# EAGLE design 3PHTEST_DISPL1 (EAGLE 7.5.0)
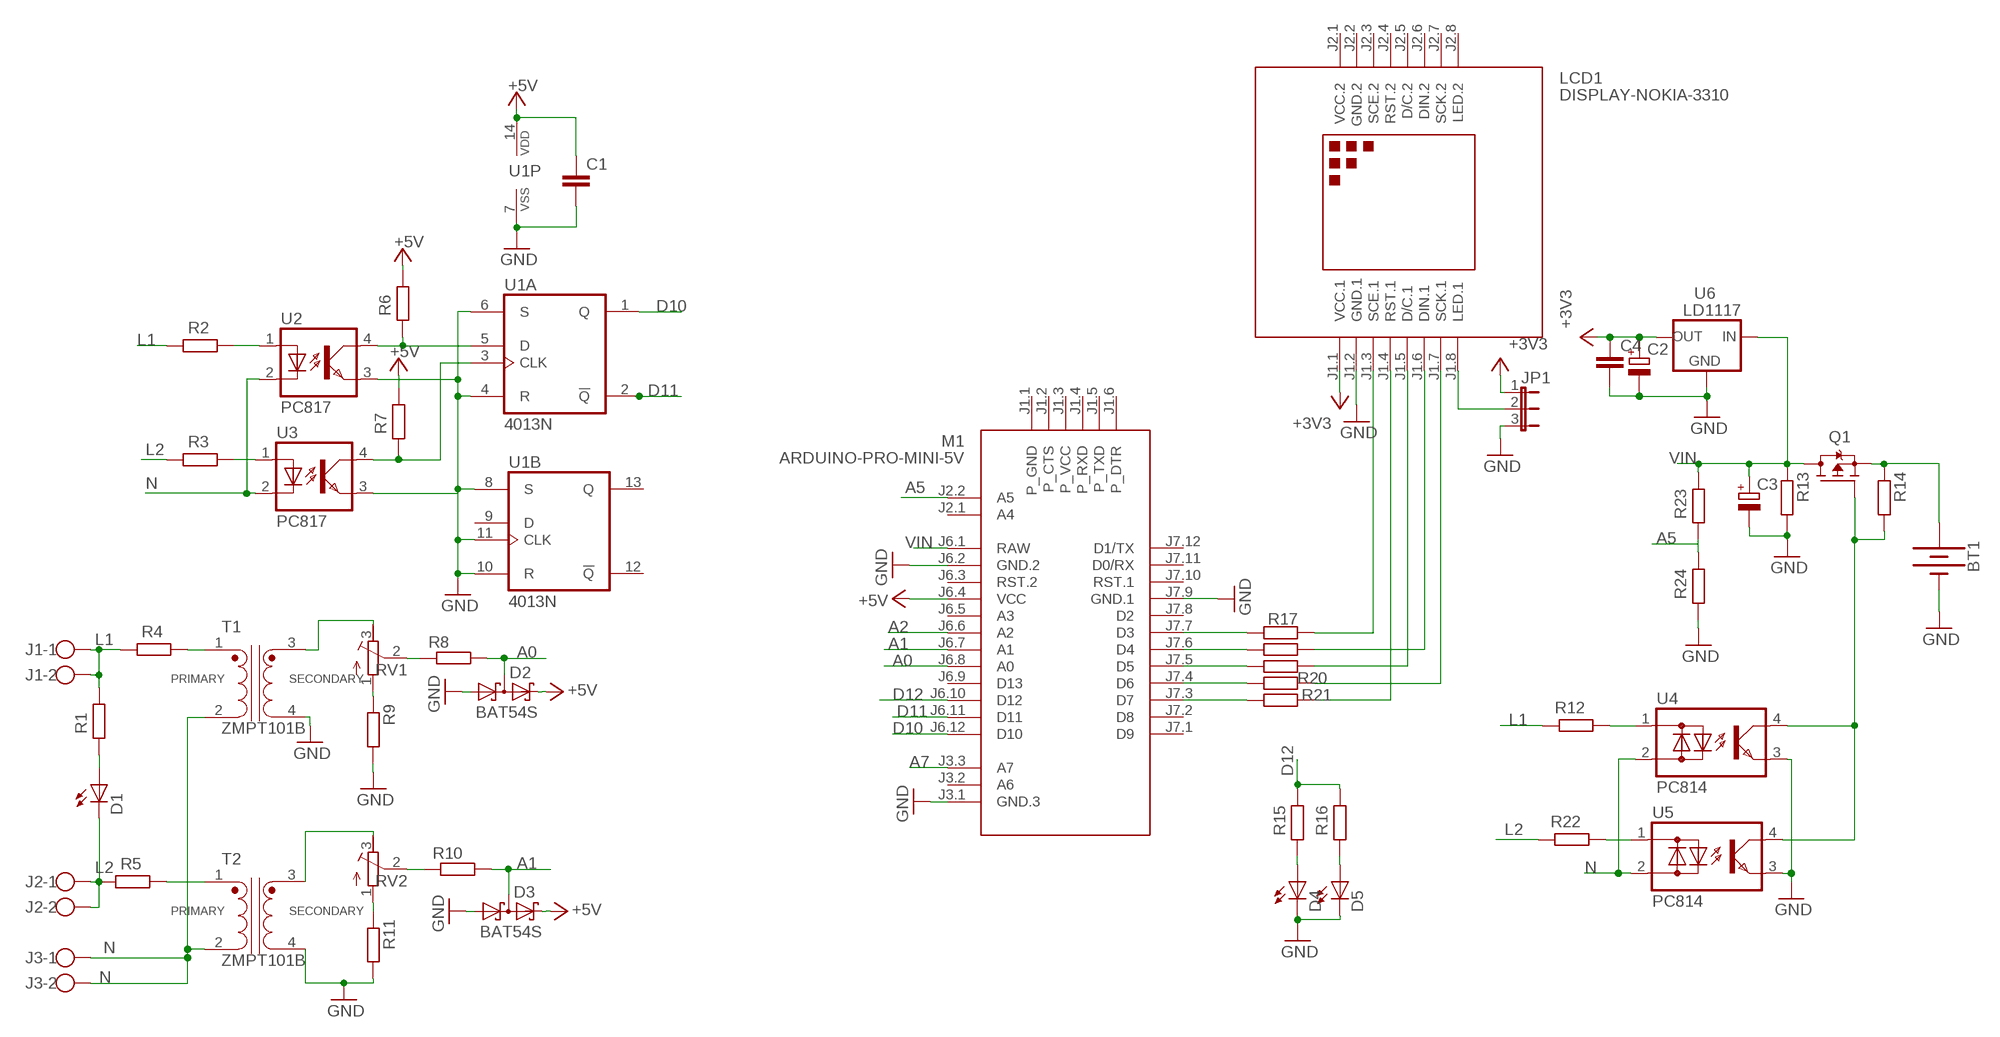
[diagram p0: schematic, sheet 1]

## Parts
BT1  BATTERY-9V  [BATTCON_9V]
C1  C-EUC1206  [C1206]
C2  CPOL-EUSMCB  [SMC_B]
C3  CPOL-EUSMCB  [SMC_B]
C4  C-EUC1206  [C1206]
D1  LED5MM  [LED5MM]
D2  BAT54S  [SOT23]
D3  BAT54S  [SOT23]
D4  LED5MM  [LED5MM]
D5  LED5MM  [LED5MM]
J1  W237-102  [W237-102]
J2  W237-102  [W237-102]
J3  W237-102  [W237-102]
JP1  JP2E  [JP2]
LCD1  DISPLAY-NOKIA-3310  [DISPLAY-NOKIA-3310]
M1  ARDUINO-PRO-MINI-5V  ARDUINO-PRO-MINI-3.3V  [ARDUINO-PRO-MINI]
Q1  STR2P3LLH6  [SOT23]
R1  R-EU_R2512  [R2512]
R2  R-EU_R2512  [R2512]
R3  R-EU_R2512  [R2512]
R4  R-EU_R2512  [R2512]
R5  R-EU_R2512  [R2512]
R6  R-EU_R1206  [R1206]
R7  R-EU_R1206  [R1206]
R8  R-EU_R1206  [R1206]
R9  R-EU_R1206  [R1206]
R10  R-EU_R1206  [R1206]
R11  R-EU_R1206  [R1206]
R12  R-EU_R2512  [R2512]
R13  R-EU_R1206  [R1206]
R14  R-EU_R1206  [R1206]
R15  R-EU_R1206  [R1206]
R16  R-EU_R1206  [R1206]
R17  R-EU_R1206  [R1206]
R18  R-EU_R1206  [R1206]
R19  R-EU_R1206  [R1206]
R20  R-EU_R1206  [R1206]
R21  R-EU_R1206  [R1206]
R22  R-EU_R2512  [R2512]
R23  R-EU_R1206  [R1206]
R24  R-EU_R1206  [R1206]
RV1  R-TRIMM64W  [RTRIM64W]
RV2  R-TRIMM64W  [RTRIM64W]
T1  ZMPT101B  [XFMR_ZMPT101B]
T2  ZMPT101B  [XFMR_ZMPT101B]
U1  4013N  [DIL14]
U2  PC817  [DIL04]
U3  PC817  [DIL04]
U4  PC814  [DIL04]
U5  PC814  [DIL04]
U6  LD1117  [SOT223]

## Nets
+3V3: C2.+ C4.1 JP1.1 LCD1.J1.1(VCC.1) U6.2(OUT)
+5V: C1.1 D2.2(C2) D3.2(C2) M1.J6.4(VCC) R6.1 R7.1 U1.14(P:VDD)
A0: D2.3(C1A2) M1.J6.8(A0) R8.2
A1: D3.3(C1A2) M1.J6.7(A1) R10.2
A2: M1.J6.6(A2)
A5: M1.J2.2(A5) R23.2 R24.1
A7: M1.J3.3(A7)
D10: M1.J6.12(D10) U1.1(A:Q)
D11: M1.J6.11(D11) U1.2(A:!Q)
D12: M1.J6.10(D12) R15.1 R16.1
GND: BT1.- C1.2 C2.- C3.- C4.2 D2.1(A1) D3.1(A1) D4.K(C) D5.K(C) JP1.3 LCD1.J1.2(GND.1) M1.J3.1(GND.3) M1.J6.2(GND.2) M1.J7.9(GND.1) R9.2 R11.2 R13.2 R24.2 T1.4 T2.4 U1.4(A:R) U1.6(A:S) U1.7(P:VSS) U1.8(B:S) U1.10(B:R) U1.11(B:CLK) U2.3(EMIT) U3.3(EMIT) U4.3(E) U5.3(E) U6.1(GND)
L1: J1.1 J1.2 R1.1 R2.2 R4.2 R12.2
L2: D1.K(C) J2.1 J2.2 R3.2 R5.2 R22.2
N: J3.1 J3.2 T1.2 T2.2 U2.2(C) U3.2(C) U4.2(AC2) U5.2(AC2)
N$1: BT1.+ Q1.3(S) R14.1
N$2: Q1.2(G) R14.2 U4.4(C) U5.4(C)
N$3: LCD1.J1.4(RST.1) R21.1
N$4: M1.J7.7(D3) R17.2
N$5: M1.J7.6(D4) R18.2
N$6: LCD1.J1.6(DIN.1) R18.1
N$7: M1.J7.3(D7) R21.2
N$8: LCD1.J1.7(SCK.1) R20.1
N$9: LCD1.J1.3(SCE.1) R17.1
N$10: LCD1.J1.5(D/C.1) R19.1
N$11: M1.J7.5(D5) R19.2
N$12: M1.J7.4(D6) R20.2
N$13: JP1.2 LCD1.J1.8(LED.1)
N$14: R12.1 U4.1(AC1)
N$15: R22.1 U5.1(AC1)
N$16: R9.1 RV1.1(A)
N$17: R4.1 T1.1
N$18: RV1.3(E) T1.3
N$19: R11.1 RV2.1(A)
N$20: R5.1 T2.1
N$21: RV2.3(E) T2.3
N$22: D1.A R1.2
N$23: R2.1 U2.1(A)
N$24: R3.1 U3.1(A)
N$25: R6.2 U1.5(A:D) U2.4(COL)
N$26: R7.2 U1.3(A:CLK) U3.4(COL)
N$27: D4.A R15.2
N$28: D5.A R16.2
N$29: R8.1 RV1.2(S)
N$32: R10.1 RV2.2(S)
VIN: C3.+ M1.J6.1(RAW) Q1.1(D) R13.1 R23.1 U6.3(IN)
Unconnected: LCD1.J2.3(SCE.2) LCD1.J2.4(RST.2) LCD1.J2.5(D/C.2) LCD1.J2.6(DIN.2) LCD1.J2.7(SCK.2) LCD1.J2.8(LED.2) M1.J1.1(P_GND) M1.J1.2(P_CTS) M1.J1.3(P_VCC) M1.J1.4(P_RXD) M1.J1.5(P_TXD) M1.J1.6(P_DTR) M1.J2.1(A4) M1.J3.2(A6) M1.J6.3(RST.2) M1.J6.5(A3) M1.J6.9(D13) M1.J7.1(D9) M1.J7.2(D8) M1.J7.8(D2) M1.J7.10(RST.1) M1.J7.11(D0/RX) M1.J7.12(D1/TX) U1.9(B:D) U1.12(B:!Q) U1.13(B:Q)

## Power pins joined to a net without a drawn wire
GND.2: LCD1.J2.2(GND.2)
VCC.2: LCD1.J2.1(VCC.2)

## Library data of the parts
BT1 = SparkFun-Batteries:BATTERY: Battery - Single Cell; PROD_ID: BATT-10855
C1 C4 = rcl:C-EU: CAPACITOR, European symbol
C2 C3 = rcl:CPOL-EU: POLARIZED CAPACITOR, European symbol
D1 D4 D5 = led:LED: LED
D2 D3 = diode:BAT54S: Schottky Diodes Pin connection corrected 2011-05-04 Source: Fairchild .. BAT54.pdf
J1-J3 = con-wago-500:W237-102: WAGO SCREW CLAMP; MPN: 237-102; OC_FARNELL: unknown; OC_NEWARK: 70K9898
JP1 = jumper:JP2E: JUMPER
LCD1 = diy-modules:DISPLAY-NOKIA-3310: 84x48 Dot Matrix LCD Module based on Nokia 3310 display More details available here: https://arduinoandsoftware.wordpress.com/2012/12/30/nokia-33105110-3-3v-display-with-5v-arduino/
M1 = diy-modules:ARDUINO-PRO-MINI-*: Arduino Pro Mini and compatible devices More details available here: https://www.arduino.cc/en/Main/ArduinoBoardProMini Click here to find device on ebay.com
Q1 = transistor-fet:STR2P3LLH6
R1-R24 = rcl:R-EU_: RESISTOR, European symbol
RV1 RV2 = rcl:R-TRIMM: Trimm resistor
T1 T2 = ZMPT101B:ZMPT101B: Check availability; AVAILABILITY: Not in stock; CHECK_PRICES: https://www.snapeda.com/parts/ZMPT101B/Qingxian+Zeming+Langxi+Electronic/view-part/?ref=eda; DESCRIPTION: Current-type Voltage Transformer; MF: Qingxian Zeming Langxi Electronic; MP: ZMPT101B; PACKAGE: None; PRICE: None; SNAPEDA_LINK: https://www.snapeda.com/parts/ZMPT101B/Qingxian+Zeming+Langxi+Electronic/view-part/?ref=snap
U1 = 40xx:4013: Dual D FLIP FLOP, set/reset
U2 U3 = optocoupler:PC817: SHARP OPTO COUPLER; MPN: PC817X4J000F; OC_FARNELL: 9707727; OC_NEWARK: 97K7059
U4 U5 = optocoupler:PC814: SHARP OPTO COUPLER; OC_FARNELL: 9707662; OC_NEWARK: unknown
U6 = v-reg:LD1117

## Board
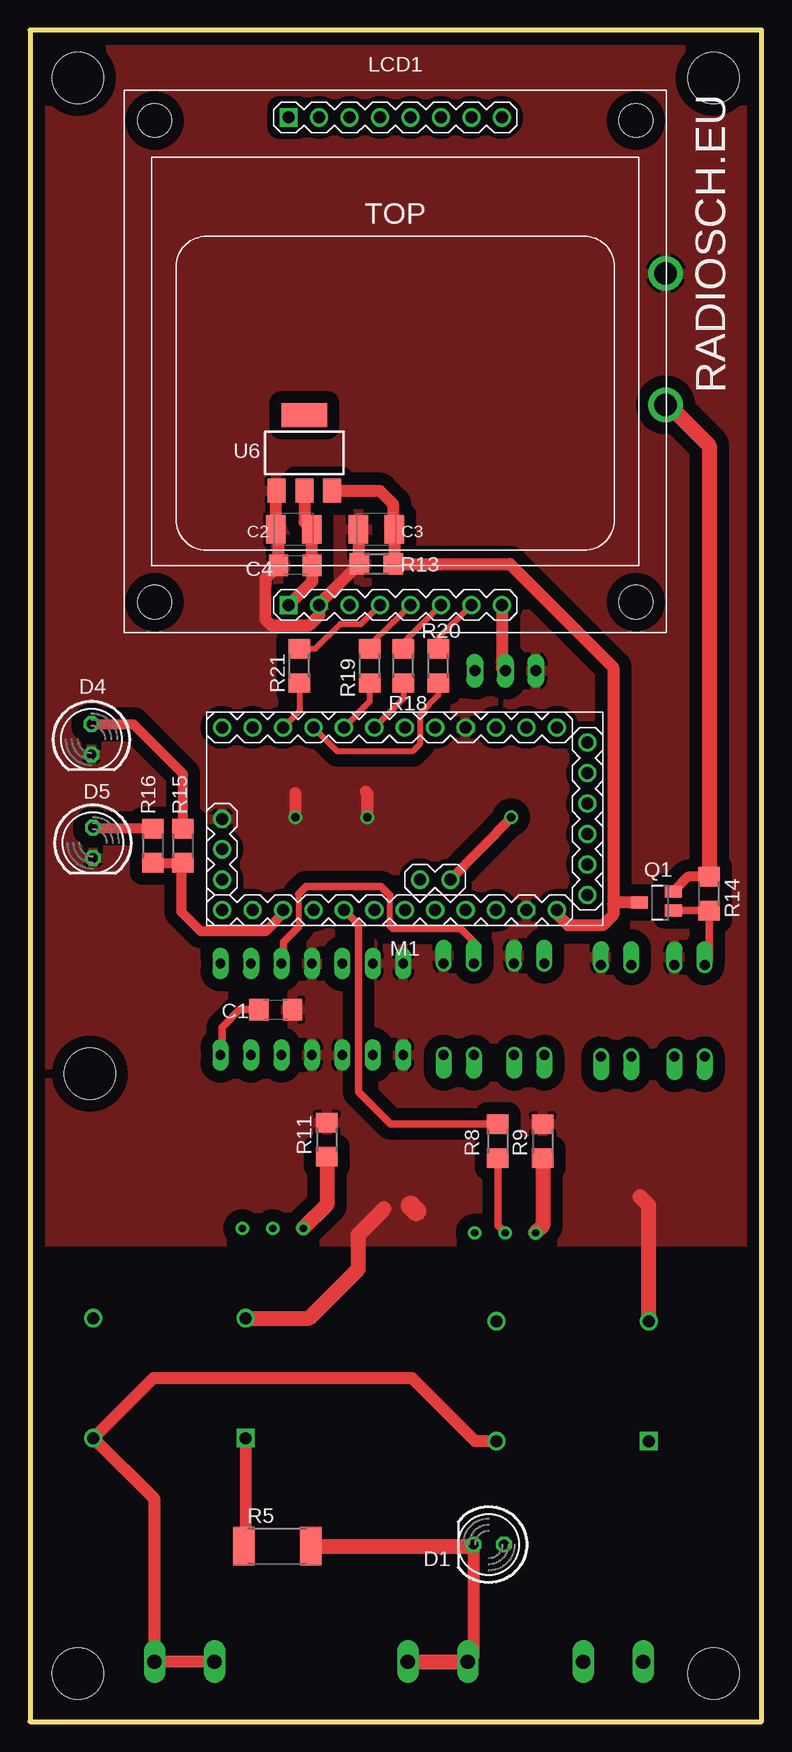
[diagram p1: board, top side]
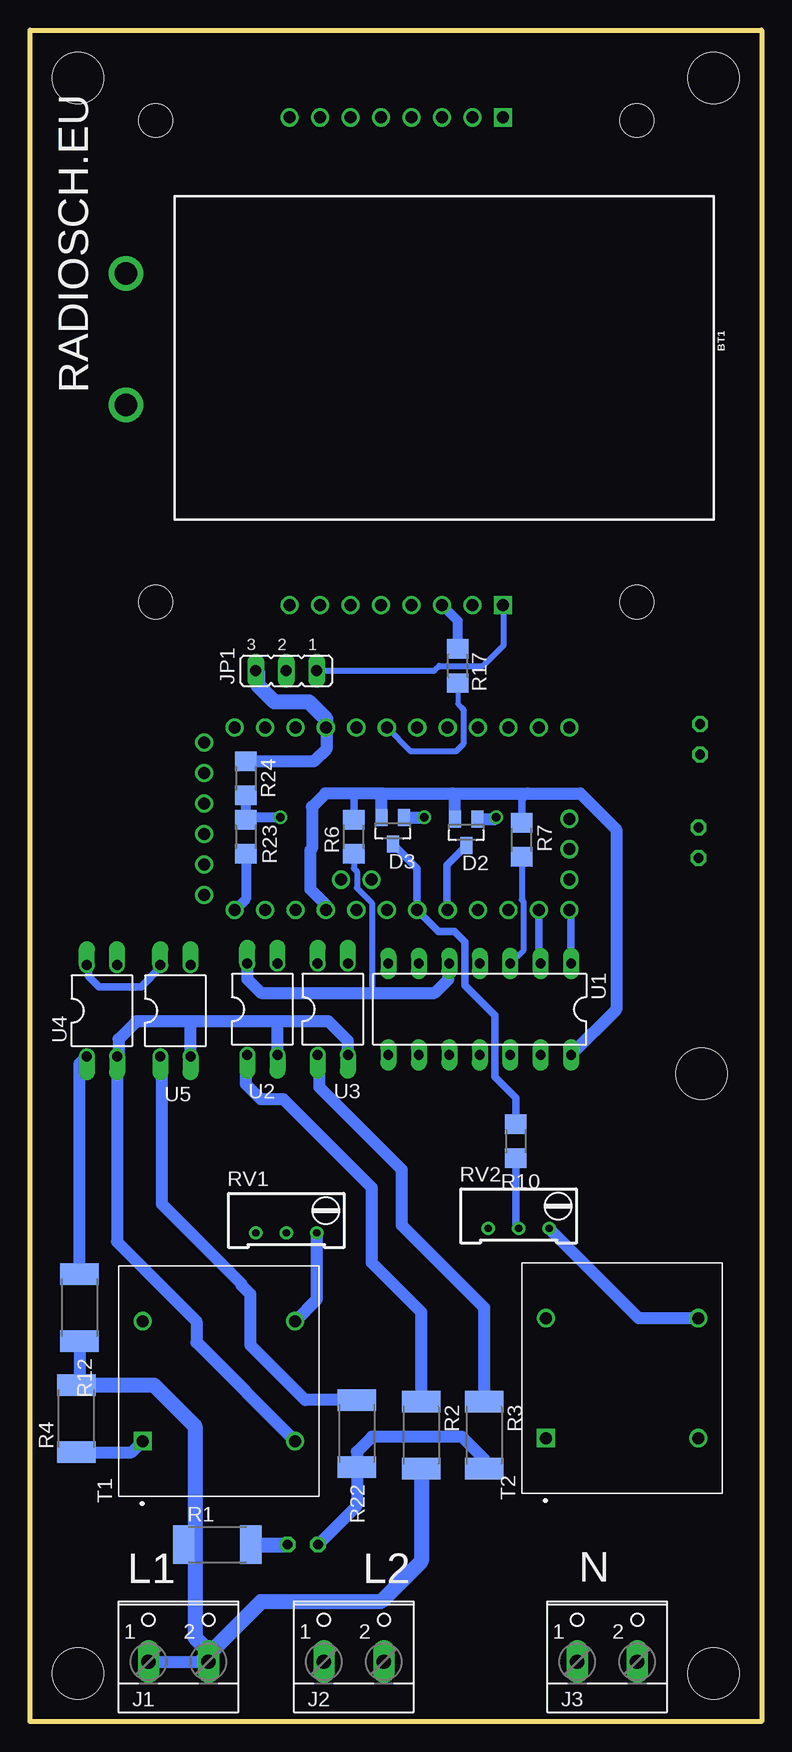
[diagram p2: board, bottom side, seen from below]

Size 61 x 141 mm. Coordinates in mm from the lower left corner, seen from the top.
Outline: 0,0 61,0 61,141 0,141 0,0
Copper layers (1*16): Top 0.035mm / dielectric 1.5mm / Bottom 0.035mm
Design rules "default": minimum track width 10mil, minimum drill 24mil, track to track 8mil, track to pad 8mil, pad to pad 8mil, via to via 8mil, smd to smd 8mil, copper to edge 40mil, drill to drill 8mil, minimum pad ring 10mil, minimum via ring 8mil, stop-mask expansion 4mil, vias tented up to drill 0mil, thermal gap 10mil
Holes 4.3 mm at 5,54 57,4 4,137 4,4 57,137

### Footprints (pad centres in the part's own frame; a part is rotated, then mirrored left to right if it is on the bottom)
BATTCON_9V = drill 1.905: + -4,-1; - -4,-11.954
C1206 = smd 1.6 x 1.8: 1 -1.4,0; 2 1.4,0
SMC_B = smd 1.6 x 2.4: + -1.5,0; - 1.5,0
LED5MM = drill 0.813 octagon: A -1.27,0; K 1.27,0
SOT23 = smd 1 x 1.4: 1 -0.95,-1.1; 2 0.95,-1.1; 3 0,1.1
W237-102 = drill 1.194 long: 1 -2.5,-1.27; 2 2.5,-1.27
JP2 = drill 0.914 long: 1 -2.54,0; 2 0,0; 3 2.54,0
DISPLAY-NOKIA-3310 = drill 1 square: J1.1 -8.89,-20.32; J2.1 -8.89,20.32 | drill 1: J1.2 -6.35,-20.32; J1.3 -3.81,-20.32; J1.4 -1.27,-20.32; J1.5 1.27,-20.32; J1.6 3.81,-20.32; J1.7 6.35,-20.32; J1.8 8.89,-20.32; J2.2 -6.35,20.32; J2.3 -3.81,20.32; J2.4 -1.27,20.32; J2.5 1.27,20.32; J2.6 3.81,20.32; J2.7 6.35,20.32; J2.8 8.89,20.32 | hole 2.8: -20.066,-20.066; 20.066,-20.066; 20.066,20.066; -20.066,20.066
ARDUINO-PRO-MINI = drill 1: J1.1 -15.24,6.35; J1.2 -15.24,3.81; J1.3 -15.24,1.27; J1.4 -15.24,-1.27; J1.5 -15.24,-3.81; J1.6 -15.24,-6.35; J2.1 -1.27,5.08; J2.2 -3.81,5.08; J3.1 15.24,0; J3.2 15.24,2.54; J3.3 15.24,5.08; J6.1 -12.7,7.62; J6.2 -10.16,7.62; J6.3 -7.62,7.62; J6.4 -5.08,7.62; J6.5 -2.54,7.62; J6.6 0,7.62; J6.7 2.54,7.62; J6.8 5.08,7.62; J6.9 7.62,7.62; J6.10 10.16,7.62; J6.11 12.7,7.62; J6.12 15.24,7.62; J7.1 15.24,-7.62; J7.2 12.7,-7.62; J7.3 10.16,-7.62; J7.4 7.62,-7.62; J7.5 5.08,-7.62; J7.6 2.54,-7.62; J7.7 0,-7.62; J7.8 -2.54,-7.62; J7.9 -5.08,-7.62; J7.10 -7.62,-7.62; J7.11 -10.16,-7.62; J7.12 -12.7,-7.62
SOT23' = smd 1 x 1.4: 1 0,1.735; 2 -0.632,-1.1; 3 0.95,-1.1
R2512 = smd 1.8 x 3.2: 1 -2.8,0; 2 2.8,0
R1206 = smd 1.6 x 1.803: 1 -1.422,0; 2 1.422,0
RTRIM64W = drill 0.61: 1 1.27,-2.54; 2 1.27,0; 3 1.27,2.54
XFMR_ZMPT101B = drill 1 square: 1 -5,6.35 | drill 1: 2 -5,-6.35; 3 5,-6.35; 4 5,6.35
DIL14 = drill 0.813 long: 1 -7.62,-3.81; 2 -5.08,-3.81; 3 -2.54,-3.81; 4 0,-3.81; 5 2.54,-3.81; 6 5.08,-3.81; 7 7.62,-3.81; 8 7.62,3.81; 9 5.08,3.81; 10 2.54,3.81; 11 0,3.81; 12 -2.54,3.81; 13 -5.08,3.81; 14 -7.62,3.81
DIL04 = drill 0.813 offset: 1 -1.27,-3.81; 2 1.27,-3.81; 3 1.27,3.81; 4 -1.27,3.81
SOT223 = smd 1.5 x 2: 1 -2.3,-3.15; 2 0,-3.15; 3 2.3,-3.15 | smd 3.8 x 2: 4 0,3.15

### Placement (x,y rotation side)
BT1  57,108.75 180 bottom
C1  20.49,59.34 0 top
C2  22,99.38 180 top
C3  28.88,99.38 180 top
C4  22.12,96.38 180 top
D1  38.25,14.75 180 top
D2  24.62,74.12 180 bottom
D3  30.75,74.25 180 bottom
D4  5.12,81.88 270 top
D5  5.25,73.25 270 top
J1  48.62,6.25 0 bottom
J2  34,6.25 0 bottom
J3  12.88,6.25 0 bottom
JP1  39.63,87.6 180 bottom
LCD1  30.46,113.39 0 top
M1  31.25,75.25 180 top
Q1  STR2P3LLH6  [SOT23']  52.55,68.25 90 top
R1  45.38,14.75 0 bottom
R2  28.38,23.88 270 bottom
R3  23.12,23.88 270 bottom
R4  57.12,25.25 90 bottom
R5  20.62,14.62 0 top
R6  34,73.75 270 bottom
R7  20,73.5 270 bottom
R8  39,48.38 90 top
R9  42.75,48.38 90 top
R10  20.5,48.38 90 bottom
R11  24.75,48.5 90 top
R12  56.88,34.5 270 bottom
R13  28.88,96.5 180 top
R14  56.62,69 270 top
R15  12.75,73 90 top
R16  10.25,73 90 top
R17  25.33,88 270 bottom
R18  31.12,88 270 top
R19  28.33,88 270 top
R20  34.03,88 270 top
R21  22.46,88 270 top
R22  33.75,24 270 bottom
R23  43,73.75 90 bottom
R24  43,78.62 90 bottom
RV1  39.62,42 270 bottom
RV2  20.25,42.38 270 bottom
T1  45.25,28.38 90 bottom
T2  11.62,28.62 90 bottom
U1  23.5,59.38 180 bottom
U2  41.62,59.38 0 bottom
U3  35.75,59.38 0 bottom
U4  55,59.25 0 bottom
U5  48.88,59.25 0 bottom
U6  22.88,105.75 0 top

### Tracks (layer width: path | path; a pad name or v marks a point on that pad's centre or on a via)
+3V3
  Top 1.016: U6.2 22.88,100 C2.+ 23.52,99.35 C4.1 23.52,95.03 LCD1.J1.1
  Bottom 0.5: JP1.1 27.27,87.6 26.88,88 23.25,88 21.5,89.75 21.5,93 LCD1.J1.1
+5V
  Top 0.61: C1.1 17.46,59.34 16,57.88 16,55.69 U1.14
  Bottom 0.61: R6.1 34,77.12 33.75,77.38 | R7.1 20,76.88 19.5,77.38
  Bottom 1.016: M1.J6.4 36.33,68.08 37.62,69.38 37.62,72.62 37.5,72.75 37.5,76.25 36.38,77.38 33.75,77.38 31.62,77.38 | 31.62,77.38 25.75,77.38 | 25.75,77.38 19.5,77.38 15.12,77.38 12.12,74.38 12.12,59.32 U1.14 | D3.2 31.7,77.3 31.62,77.38 | D2.2 25.57,77.2 25.75,77.38
A0
  Top 0.61: R8.2 30.08,49.8 27.38,52.5 27.38,66.42 M1.J6.8
  Bottom 0.61: M1.J6.8 26.25,67.71 26.25,71.4 D2.3
A1
  Bottom 0.61: R10.2 20.5,52 22.25,53.75 22.25,58.88 24.75,61.38 24.75,65 25.62,65.88 26.95,65.88 M1.J6.7 28.71,71.11 D3.3
A5  (via drill 0.7)
  Top 0.813: M1.J2.2 35.06,70.19 v40.12,75.38
  Bottom 0.813: R24.1 R23.2 42.8,75.38 v40.12,75.38
D10
  Bottom 0.61: U1.1 15.88,67.5 M1.J6.12
D11
  Bottom 0.61: M1.J6.11 18.55,63.31 U1.2
D12
  Top 0.813: R16.1 R15.1 12.62,71.45 12.62,67.5 14.25,65.88 19.62,65.88 21.09,67.34 M1.J6.10
GND  (via drill 0.7)
  Top 1.016: U6.1 20.5,102.53 C2.- 20.73,99.15 C4.2 19.62,95.28 19.62,91.88 20.12,91.38 23.25,91.38 24.11,92.23 LCD1.J1.2 24.11,93.16 R13.2 27.38,96.58 C3.- | v28.12,75.38 28.12,77.38 28,77.5 | v22.12,75.38 22.12,77.38
  Top 1.27: T1.4 51.6,43.02 50.88,43.75 | T2.4 23.25,33.62 27.38,37.75 27.38,40.62 29.5,42.75
  Top 1.676: 32.23,42.52 31.75,43
  Bottom 1.016: D3.1 28.15,75.35 v28.12,75.38 | D2.1 22.27,75.22 v22.12,75.38 | R24.2 37.33,80.05 36.25,81.12 36.25,82.79 M1.J7.9
  Bottom 1.27: M1.J7.9 36.33,83.58 37.75,85 40.62,85 42,86.38 42,87.42 JP1.3
  pour Top (isolate 1.016): 1,141 60,141 60,40 1,40
L1
  Bottom 1.016: J1.1 46.75,4.98 J1.2 | R12.2 56.88,28.3 R4.2
  Bottom 1.27: R2.2 28.38,13.38 31.75,10 41.73,10 45.99,5.74 | 45.99,5.74 46.75,4.98 | R4.2 50.67,28.05 47.25,24.62 47.25,14.75 | 47.25,14.75 47.25,7 45.99,5.74 | R1.1 47.25,14.75
L2
  Top 1.016: 36.85,14.88 D1.K 36.98,5.46 J2.1
  Top 1.27: J2.2 J2.1 | R5.2 36.85,14.62 D1.K
  Bottom 1.016: R3.2 23.12,21.88 25,23.75 32.5,23.75 33.75,22.5 R22.2 33.75,17.98 D1.K
N
  Top 1.016: T1.2 37.12,23.38 31.88,28.62 10.28,28.62 T2.2 10.38,18.52 J3.2 J3.1
  Bottom 1.016: U3.2 34.48,56.73 36.12,58.38 40.62,58.38 | 40.62,58.38 47.88,58.38 | 47.88,58.38 52.12,58.38 53.62,56.88 53.62,55.55 U4.2 53.73,39.98 47.12,33.38 47.12,31.6 T1.2 | U2.2 40.35,57.73 40.38,57.75 40.38,58.12 40.62,58.38 | U5.2 47.6,58.1 47.88,58.38
N$1
  Top 0.813: R14.1 54.86,70.42 Q1.3
  Top 1.27: BT1.+ 53.25,109.75 56.62,106.38 R14.1
N$2
  Top 0.61: U4.4 56.62,63.41 R14.2 56.58,67.62 Q1.2
  Bottom 0.61: U5.4 50.15,62.85 51.75,61.25 55.25,61.25 56.12,62.12 56.12,62.91 U4.4
N$3
  Top 0.5: R21.1 23.79,89.42 25.88,91.5 27.62,91.5 LCD1.J1.4
N$4
  Bottom 0.406: R17.2 25.33,84.83 25,84.5
  Bottom 0.5: 25,84.5 24.88,84.38 24.88,81.5 25.5,80.88 29.25,80.88 M1.J7.7
N$5
  Top 0.5: R18.2 31.12,85.28 M1.J7.6
N$6
  Top 0.5: R18.1 31.12,89.92 LCD1.J1.6
N$7
  Top 0.5: R21.2 22.46,84.25 M1.J7.3
N$8
  Top 0.5: R20.1 34.03,90.3 LCD1.J1.7
N$9
  Bottom 0.813: R17.1 25.33,91.75 LCD1.J1.3
N$10
  Top 0.5: R19.1 28.33,89.7 30.25,91.62 30.29,91.62 LCD1.J1.5
N$11
  Top 0.5: R19.2 28.33,85.03 M1.J7.5
N$12
  Top 0.5: R20.2 34.03,85.53 32.5,84 32.5,81.5 31.88,80.88 25.62,80.88 M1.J7.4
N$13
  Top 1.016: LCD1.J1.8 39.35,87.89 JP1.2
N$14
  Bottom 1.016: R12.1 56.88,54.84 U4.1
N$15
  Bottom 1.016: R22.1 38.05,26.8 42.62,31.38 42.62,35.62 43.38,36.38 43.38,36.5 50,43.12 50,55.3 U5.1
N$16
  Top 1.27: R9.1 42.75,41.31 RV1.1
N$17
  Bottom 1.016: R4.1 52.52,22.45 T1.1
N$18
  Bottom 1.016: RV1.3 37.09,35.19 T1.3
N$19
  Top 1.27: R11.1 24.75,43.06 RV2.1
N$20
  Top 1.016: T2.1 17.98,14.78 R5.1
N$21
  Bottom 1.016: T2.3 10.23,33.62 RV2.3
N$22
  Bottom 1.27: R1.2 D1.A
N$23
  Bottom 1.016: R2.1 28.38,34.12 32.5,38.25 32.5,44.5 39.88,51.88 41.75,51.88 43,53.12 43,55.46 U2.1
N$24
  Bottom 1.016: U3.1 36.88,55.42 36.88,52.88 30,46 30,41.38 23.12,34.5 R3.1
N$25
  Bottom 0.5: R6.2 34,71.12 33.75,70.88 33.75,69.5 32.5,68.25 32.5,60.75
  Bottom 1.016: U2.4 42.9,61.9 41.75,60.75 32.5,60.75 27.25,60.75 26.12,61.88 26.12,63.1 U1.5
N$26
  Top 0.5: 30,66.38 30,68.88 | 22.38,69 22.38,66.25
  Top 0.61: U3.4 37.02,64.98 35.88,66.12 30.25,66.12 30,66.38 | 30,68.88 29.25,69.62 23,69.62 22.38,69 | 22.38,66.25 21.12,65 21.12,63.35 U1.3
  Bottom 0.5: R7.2 20,68.5 19.88,68.38 19.88,64.27 U1.3
N$27
  Top 0.813: R15.2 12.75,79 8.62,83.12 5.14,83.12 D4.A
N$28
  Top 0.813: R16.2 5.35,74.42 D5.A
N$29
  Top 0.61: R8.1 39,41.35 RV1.2
N$32
  Bottom 0.61: R10.1 20.5,41.35 RV2.2
VIN
  Top 1.016: U6.3 29.15,102.6 30.25,101.5 30.25,99.5 C3.+ 30.38,96.58 R13.1 40,96.5 48.62,87.88 48.62,68.12 | 48.62,68.12 48.62,67.25 47.75,66.38 44.88,66.38 44.12,67.12 44.12,67.45 M1.J6.1 | Q1.1 48.76,68.25 48.62,68.12
  Bottom 0.813: R23.1 43,68.58 M1.J6.1

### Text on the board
tPlace: RADIOSCH.EU
bPlace: RADIOSCH.EU | N | L2 | L1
